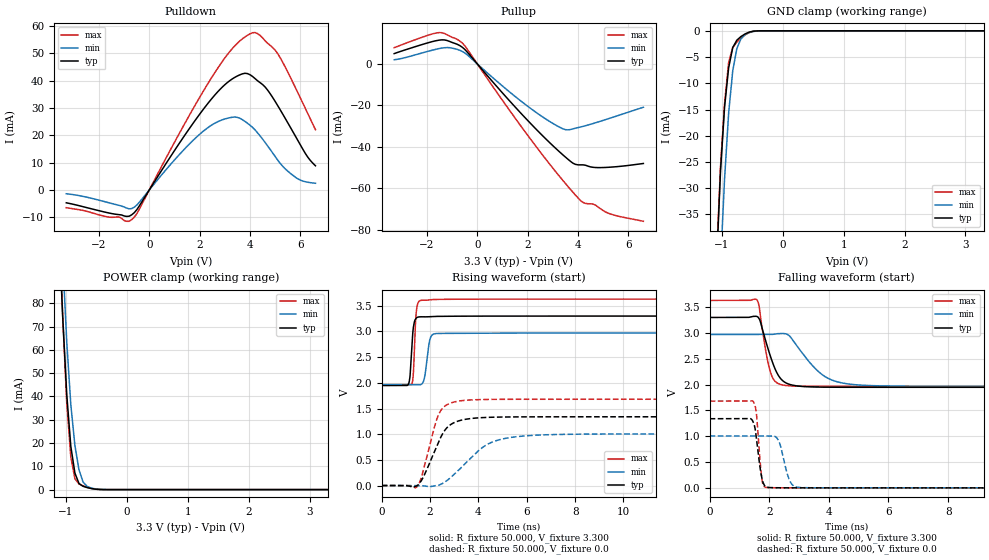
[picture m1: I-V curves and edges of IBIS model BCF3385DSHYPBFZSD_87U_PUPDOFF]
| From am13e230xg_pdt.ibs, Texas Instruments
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|   Model BCF3385DSHYPBFZSD_87U_PUPDOFF
[Model] BCF3385DSHYPBFZSD_87U_PUPDOFF
Model_type I/O
Polarity   Non-Inverting
Enable   Active-Low
Vinl =  0.990V
Vinh =  2.310V
Vmeas =  1.650V
C_comp   0.589pF   0.544pF   0.642pF
[Model Spec]
Vinh   2.310V   2.079V   2.541V
Vinl   0.990V   0.891V   1.089V
Vmeas   1.650V   1.485V   1.815V
[Temperature Range]   25.000   0.155k   -40.000
[Voltage Range]   3.300V   2.970V   3.630V
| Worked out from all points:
|   slope of the pulldown table from 0 to 0.495 V, typ, clamps not added: 68.5 ohm
|   slope of the pullup table from 0 to 0.495 V, typ, clamps not added: 70.6 ohm
|   GND clamp passes 1 mA (typ) near -0.67 V on its own axis
|   POWER clamp passes 1 mA (typ) near -0.67 V on its own axis
|   rising waveform, R_fixture 50.000, V_fixture 3.300: 20-80 % time 110ps typ, 165ps min, 91.9ps max; typ from 1.95 V to 3.3 V
|   rising waveform, R_fixture 50.000, V_fixture 0.0: 20-80 % time 779ps typ, 1.42ns min, 574ps max; typ from 0 V to 1.34 V
|   falling waveform, R_fixture 50.000, V_fixture 3.300: 20-80 % time 475ps typ, 935ps min, 302ps max; typ from 3.3 V to 1.95 V
|   falling waveform, R_fixture 50.000, V_fixture 0.0: 20-80 % time 180ps typ, 263ps min, 136ps max; typ from 1.34 V to 0 V
[Pulldown]
|Voltage   I(typ)   I(min)   I(max)
-3.3V     -4.738mA   -1.439mA   -6.529mA
-700mV    -9.134mA   -6.846mA   -10.9mA
-400mV    -5.894mA   -4.558mA   -7.098mA
1.4V      19.9mA     14.97mA    24.17mA
2.4V      32.5mA     23.26mA    40.01mA
3.4V      41.22mA    26.67mA    52.78mA
3.8V      42.69mA    25.06mA    56.01mA
4.1V      41.52mA    22.89mA    57.53mA
4.6V      37.66mA    17.36mA    54.58mA
5.1V      30.85mA    10.91mA    49.89mA
5.9V      18.1mA     4.028mA    35.58mA
6.6V      8.813mA    2.416mA    22.04mA
[Pullup]
|Voltage   I(typ)   I(min)   I(max)
-3.3V     4.951mA    1.968mA    7.808mA
-1.5V     11.48mA    7.414mA    15.11mA
-700mV    8.858mA    6.582mA    11.1mA
-400mV    5.719mA    4.386mA    7.142mA
2V        -27.27mA   -20.43mA   -34.44mA
3.5V      -44.98mA   -31.75mA   -57.71mA
3.9V      -48.52mA   -31.06mA   -63.34mA
4.2V      -48.76mA   -30.19mA   -66.89mA
4.6V      -49.94mA   -28.81mA   -67.71mA
4.9V      -50.09mA   -27.68mA   -69.99mA
5.4V      -49.78mA   -25.73mA   -72.89mA
6.6V      -48.1mA    -20.94mA   -76.01mA
[GND_clamp]
|Voltage   I(typ)   I(min)   I(max)
-3.3V     -1.006A    -883.4mA   -1.272A
-1.089V   -45.1mA    -63.73mA   -44.09mA
-1.022V   -26.78mA   -44.63mA   -25.9mA
-955mV    -14.49mA   -28.18mA   -13.81mA
-888mV    -7.028mA   -15.64mA   -6.005mA
-821mV    -3.189mA   -7.628mA   -3.171mA
-754mV    -1.786mA   -3.389mA   -2.151mA
-687mV    -1.097mA   -1.538mA   -1.399mA
-620mV    -601.7uA   -747.3uA   -782.8uA
-486mV    -70.11uA   -129.5uA   -99.51uA
-352mV    -1.527uA   -8.942uA   -1.719uA
3.3V      0A         0A         0A
[POWER_clamp]
|Voltage   I(typ)   I(min)   I(max)
-3.3V     1.772A     2.005A     1.902A
-1.122V   114.9mA    142.9mA    120.1mA
-1.055V   74.53mA    99.87mA    74.96mA
-988mV    40.92mA    63.48mA    37.22mA
-921mV    18.54mA    36.45mA    14.02mA
-854mV    7.11mA     18.97mA    4.658mA
-787mV    2.624mA    8.509mA    2.397mA
-720mV    1.421mA    3.258mA    1.612mA
-653mV    867.1uA    1.356mA    992.6uA
-586mV    464.5uA    677.9uA    496.7uA
-385mV    10.92uA    45.23uA    6.451uA
3.3V      0A         0A         0A
[Ramp]
| variable   typ   min   max
dV/dt_r   0.803/0.779n   0.603/1.418n   1.008/0.574n
dV/dt_f   0.812/0.475n   0.602/0.935n   1.000/0.302n
R_load = 50.000
[Rising Waveform]
R_fixture= 50.000
V_fixture= 3.300
V_fixture_min= 2.970
V_fixture_max= 3.630
|time   V(typ)   V(min)   V(max)
0s        1.947V     1.966V     1.964V
1.09ns    1.964V     1.966V     1.965V
1.173ns   2.148V     1.966V     1.963V
1.247ns   2.706V     1.966V     1.983V
1.305ns   3.069V     1.966V     2.16V
1.431ns   3.263V     1.965V     3.391V
1.642ns   3.286V     1.973V     3.607V
1.999ns   3.289V     2.857V     3.619V
2.245ns   3.294V     2.96V      3.624V
25ns      3.3V       2.97V      3.63V
[Rising Waveform]
R_fixture= 50.000
V_fixture= 0.0
V_fixture_min= 0.0
V_fixture_max= 0.0
|time   V(typ)   V(min)   V(max)
0s        1.247uV    1.099uV    1.11uV
1.478ns   2.237mV    651.3uV    -15.09mV
1.668ns   120.2mV    -3.627mV   205.2mV
2.197ns   681.3mV    -6.221mV   1.167V
2.376ns   875.6mV    11.23mV    1.405V
2.726ns   1.14V      107.1mV    1.581V
3.219ns   1.264V     317.4mV    1.648V
4.459ns   1.329V     823.6mV    1.677V
6.109ns   1.338V     973.1mV    1.68V
25ns      1.339V     1.005V     1.68V
[Falling Waveform]
R_fixture= 50.000
V_fixture= 3.300
V_fixture_min= 2.970
V_fixture_max= 3.630
|time   V(typ)   V(min)   V(max)
0s        3.3V       2.97V      3.63V
1.579ns   3.32V      2.97V      3.643V
1.657ns   3.281V     2.97V      3.525V
1.851ns   2.905V     2.97V      2.753V
2.055ns   2.52V      2.97V      2.215V
2.3ns     2.183V     2.986V     2.02V
2.568ns   2.03V      2.981V     1.982V
3.798ns   1.95V      2.183V     1.964V
4.918ns   1.947V     1.996V     1.964V
25ns      1.947V     1.966V     1.964V
[Falling Waveform]
R_fixture= 50.000
V_fixture= 0.0
V_fixture_min= 0.0
V_fixture_max= 0.0
|time   V(typ)   V(min)   V(max)
0s        1.339V     1.005V     1.68V
1.474ns   1.257V     1.005V     1.662V
1.571ns   953.8mV    1.005V     1.426V
1.696ns   371.1mV    1.005V     488.6mV
1.758ns   172.9mV    1.005V     144.9mV
1.921ns   14.01mV    1.005V     7.462mV
2.281ns   1.937mV    944.6mV    1.495mV
2.686ns   766.7uV    139.7mV    436.8uV
3.029ns   353.8uV    7.281mV    145.5uV
25ns      332.8nV    598.9nV    336.5nV
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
